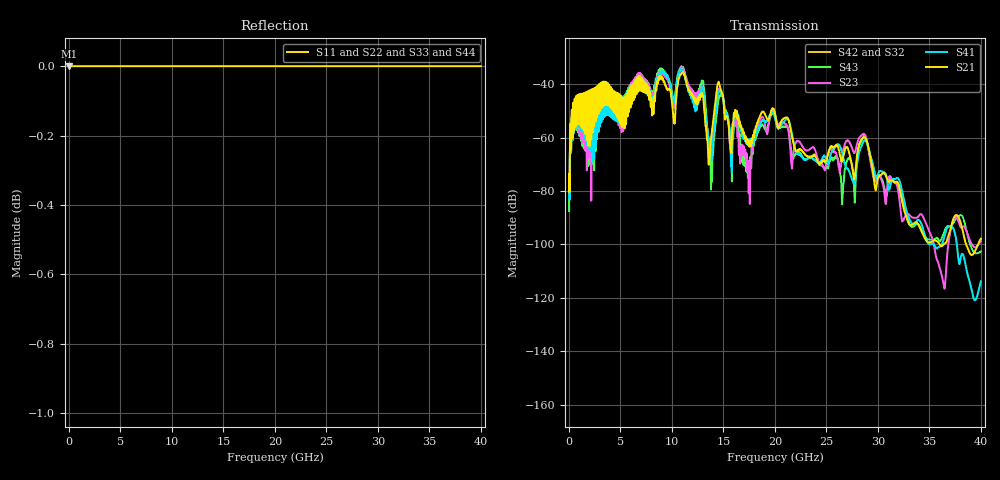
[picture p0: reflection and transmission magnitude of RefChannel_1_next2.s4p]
# GHz S RI R 50
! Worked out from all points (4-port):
!   4000 points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, 10 MHz to 40 GHz, reference 50 ohm
!   strongest paths, dB at 10 MHz, 10.01 GHz, 20.01 GHz, 30.01 GHz, 40 GHz:
!     S21: -80.4, -47.3, -51.0, -75.2, -97.9
!     S41: -81.2, -44.2, -52.5, -73.8, -113.9
!     S23: -81.6, -45.6, -51.4, -74.0, -98.8
!     S43: -87.5, -43.0, -52.8, -74.2, -102.7
!     S42: -, -, -, -, -
!     S32: -, -, -, -, -
!   lowest |S11| = 0.0 dB at 10 MHz (marker M1)
!   |S11| at or under -10 dB: nowhere
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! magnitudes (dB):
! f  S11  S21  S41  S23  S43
! 10 MHz  0.0  -80.4  -81.2  -81.6  -87.5
! 10.93 GHz  0.0  -35.8  -34.4  -33.6  -33.8
! 13.83 GHz  0.0  -59.3  -68.6  -62.5  -74.4
! 14.76 GHz  0.0  -42.4  -43.5  -42.8  -44.2
! 17.5 GHz  0.0  -63.3  -62.7  -72.2  -72.2
! 19.78 GHz  0.0  -49.0  -50.3  -49.2  -50.6
! 40 GHz  0.0  -97.9  -113.9  -98.8  -102.7
